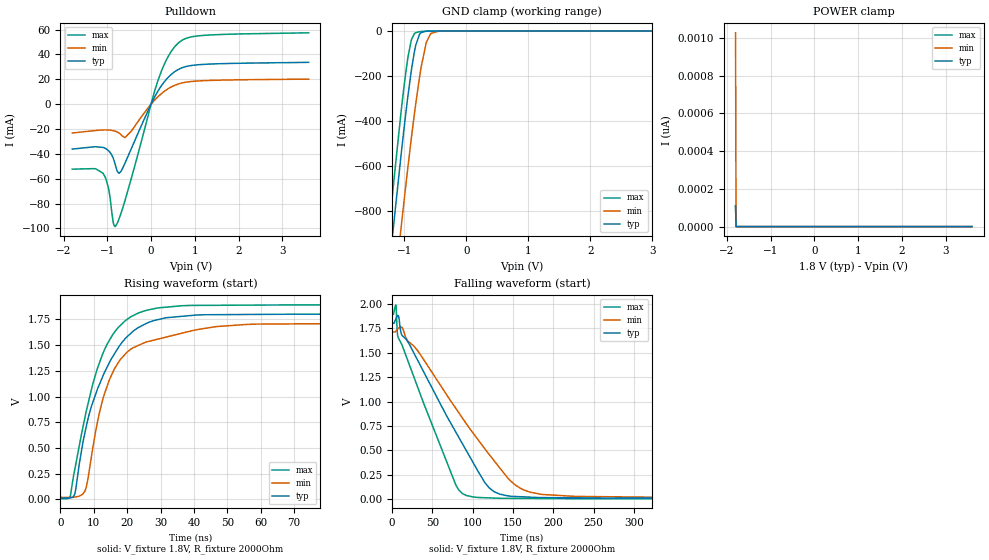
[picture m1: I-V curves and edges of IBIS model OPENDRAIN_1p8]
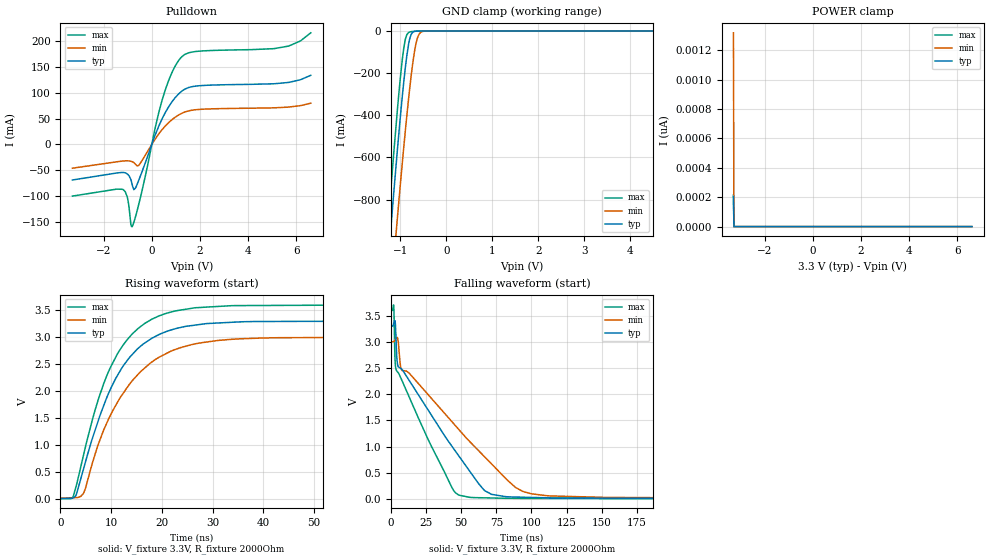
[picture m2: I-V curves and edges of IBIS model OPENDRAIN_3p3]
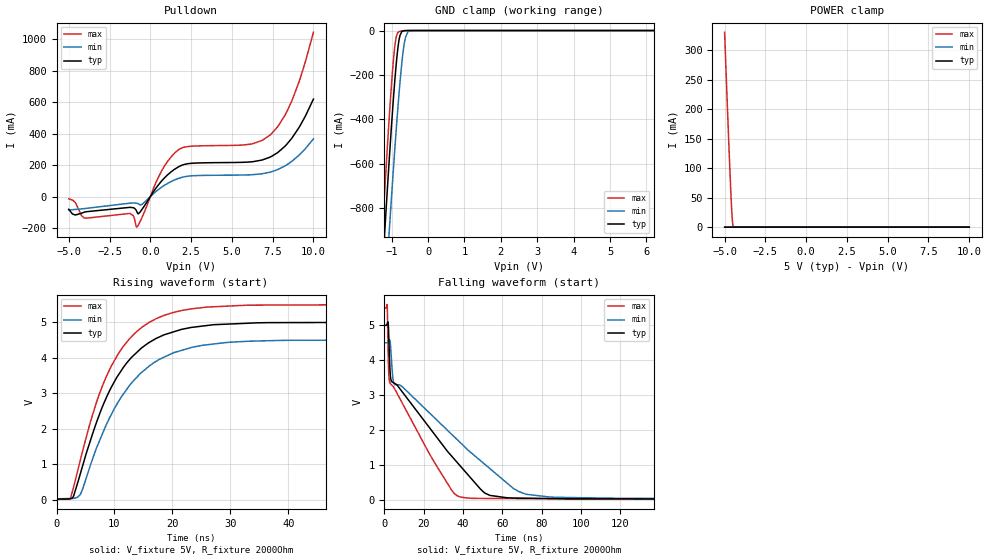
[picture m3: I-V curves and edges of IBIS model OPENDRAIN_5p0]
|Texas Instruments Incorporated
|DACx3204, Quad, 12-Bit, 10-Bit or 8-Bit, I2C Interface, Voltage/Current Output
|DACs in Tiny 3 * 3 QFN Package
[IBIS Ver]   4.1
[File name]   dac53204.ibs
[Date]   11/17/2021
[File Rev]   1.0
[Source]
| Texas Instruments Incorporated.
| Analog-eLab Design Center, HPA
| 12500 TI Blvd
| Dallas, TX -75243
[Notes]   Revision History:
| Rev 1.0: 11/17/2021
| - Initial version of the model
| - Model generated from simulations in SPECTRE
|   Model names with a trailing _1p8 contain the model for 1.8V operation.
|   Model names with a trailing _3p3 contain the model for 3.3V operation.
|   Model names with a trailing _5p0 contain the model for 5.0V operation.
| - C_comp although listed in numerical order of value are
|   obtained from varying PVT conditions. For PVT conditions for
|   each specific value refer the buffer description under
|   respective [Model]. IBIS model user is responsible for using
|   appropriate C_comp to simulate for Signal Integrity.
| - Warnings regarding combined Non-monotonicity of various models
|   have been reviewed and considered minor and can be ignored.
[Disclaimer]
| This model is designed as an aid for customers of Texas Instruments.
| TI and its licensors and suppliers make no warranties, either expressed
| or implied, with respect to this  model, including the warranties of
| merchantability or fitness for a particular purpose. The model is
| provided solely on an "as is" basis. The entire risk as to its quality
| and performance is with the customer.
| This model is subject to change without notice. Texas Instruments
| Incorporated is not responsible for updating this model.
[Copyright]
(C) Copyright 2018 Texas Instruments Incorporated.All rights reserved.
|  Component DAC53204 16-pin WQFN Package
|  Part # DAC53204
[Component]   DAC5204
[Manufacturer]  TI
[Package]   |16-pin WQFN Package
|   typ   min   max
R_pkg   0.05   0.04   0.06
L_pkg   1.0nH   0.8nH   1.2nH
C_pkg   0.2pF   0.16pF   0.24pF
[Pin]   signal_name   model_name   R_pin   L_pin   C_pin
1   FB3   NC   NA   NA   NA
2   OUT3   NC   NA   NA   NA
3   OUT2   NC   NA   NA   NA
4   FB2   NC   NA   NA   NA
5   GPIO   IO_OPENDRAIN   NA   NA   NA
6   SCL   IO_OPENDRAIN   NA   NA   NA
7   A0   IO_OPENDRAIN   NA   NA   NA
8   SDA   IO_OPENDRAIN   NA   NA   NA
9   FB1   NC   NA   NA   NA
10   OUT1   NC   NA   NA   NA
11   OUT0   NC   NA   NA   NA
12   FB0   NC   NA   NA   NA
13   CAP   NC   NA   NA   NA
14   AGND   GND   NA   NA   NA
15   VDD   POWER   NA   NA   NA
16   VREF   NC   NA   NA   NA
|   Model Selectors
[Model Selector] IO_OPENDRAIN
OPENDRAIN_1p8  1.8V   digital I/O_open_drain
OPENDRAIN_3p3  3.3V   digital I/O_open_drain
OPENDRAIN_5p0  5.0V   digital I/O_open_drain
| Models and submodels in the file (3): OPENDRAIN_1p8 (I/O_open_drain), OPENDRAIN_3p3 (I/O_open_drain), OPENDRAIN_5p0 (I/O_open_drain)
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|   OPENDRAIN_1p8 Model
[Model]   OPENDRAIN_1p8
Model_type   I/O_open_drain
Polarity   Non-Inverting
Enable   Active-Low
Vinl = 0.4
Vinh = 1.62
Vmeas = 0.9
Vref = 1.8
Cref = 2pF
Rref = 2000
|   typ   min   max
C_comp   1.258pF   1.229pF   1.287pF
[Voltage Range]   1.8   1.71   1.89
[Temperature Range]   25   125   -40
[Pullup Reference]   1.8   1.71   1.89
[Pulldown Reference]   -0   -0   0
[Power Clamp Reference]   1.8   1.71   1.89
[GND Clamp Reference]   0   0   0
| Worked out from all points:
|   slope of the pulldown table from 0 to 0.27 V, typ, clamps not added: 16.4 ohm
|   GND clamp passes 1 mA (typ) near -0.65 V on its own axis
|   falling waveform, V_fixture 1.8V, R_fixture 2000Ohm: 20-80 % time 70.5ns typ, 86.4ns min, 52.5ns max; typ from 1.8 V to 0.012 V
|   rising waveform, V_fixture 1.8V, R_fixture 2000Ohm: 20-80 % time 10.9ns typ, 9.29ns min, 9.24ns max; typ from 0.012 V to 1.8 V
[Pulldown]
|   Voltage   I(typ)   I(min)   I(max)
-1.8V     -36.15mA   -23.22mA   -52.32mA
-1.098V   -34.82mA   -20.75mA   -55.58mA
-979.2mV  -37.21mA   -20.78mA   -66.6mA
-865.8mV  -43.37mA   -21.34mA   -94.86mA
-817.2mV  -48.87mA   -21.79mA   -98.5mA
-682.2mV  -53.81mA   -24.75mA   -87.4mA
-444.6mV  -35.27mA   -21.46mA   -58.93mA
160.2mV   10.68mA    6.088mA    19.27mA
387mV     21.43mA    12.35mA    38.11mA
613.8mV   27.79mA    16.14mA    48.97mA
1.143V    31.91mA    18.82mA    55.22mA
3.6V      33.67mA    20.17mA    57.45mA
[GND Clamp]
|   Voltage   I(typ)   I(min)   I(max)
-1.8V     -2.596A    -2.851A    -2.471A
-1.433V   -1.564A    -1.858A    -1.402A
-1.201V   -928.8mA   -1.245A    -744.2mA
-1.179V   -871.1mA   -1.189A    -684.9mA
-1.055V   -548.9mA   -872.2mA   -358.3mA
-941.4mV  -281.8mA   -596mA     -112.3mA
-882mV    -162.3mA   -459.7mA   -34.2mA
-822.6mV  -68.79mA   -332mA     -7.838mA
-757.8mV  -15.19mA   -206.4mA   -2.984mA
-644.4mV  -611.1uA   -48.59mA   -607.3uA
-444.6mV  -4.804uA   -314.9uA   -3.221uA
3.6V      0A         0A         0A
[POWER Clamp]
|   Voltage   I(typ)   I(min)   I(max)
-1.8V     109.3pA    1.028nA    111pA
-1.789V   0A         0A         0A
-1.784V   0A         0A         0A
3.6V      0A         0A         0A
[Ramp]
R_load = 2000
|   typ   min   max
dV/dt_r   1.07282/1.08624e-08   1.01393/9.23116e-09   1.12988/9.2542e-09
dV/dt_f   1.07282/7.03748e-08   1.01391/8.57477e-08   1.12988/5.24625e-08
[Falling Waveform]
V_fixture = 1.8V
V_fixture_min = 1.71V
V_fixture_max = 1.89V
R_fixture = 2000Ohm
C_fixture = 0F
|   Time   V(typ)   V(min)   V(max)
0s        1.8V       1.71V      1.89V
4.646ns   1.845V     1.719V     1.988V
7.422ns   1.879V     1.748V     1.657V
12.07ns   1.68V      1.76V      1.583V
78.53ns   695.1mV    936.2mV    158mV
100.3ns   378.8mV    679.9mV    24.79mV
120.3ns   118.6mV    459.6mV    15.15mV
152.8ns   29.52mV    146.2mV    10.18mV
226.9ns   15.67mV    30.27mV    7.485mV
1.5us     11.97mV    20.15mV    6.861mV
[Rising Waveform]
V_fixture = 1.8V
V_fixture_min = 1.71V
V_fixture_max = 1.89V
R_fixture = 2000Ohm
C_fixture = 0F
|   Time   V(typ)   V(min)   V(max)
0s        11.96mV    20.12mV    6.859mV
2.913ns   14.36mV    20.15mV    27.5mV
4.236ns   47.13mV    22.99mV    281.4mV
7.365ns   652.5mV    83.69mV    800.3mV
11.76ns   1.124V     853.2mV    1.334V
15.61ns   1.385V     1.23V      1.598V
23.2ns    1.668V     1.494V     1.809V
36.28ns   1.779V     1.614V     1.882V
90.43ns   1.8V       1.71V      1.89V
1.5us     1.8V       1.71V      1.89V
|   OPENDRAIN_3p3 Model
[Model]   OPENDRAIN_3p3
Model_type   I/O_open_drain
Polarity   Non-Inverting
Enable   Active-Low
Vinl = 0.4
Vinh = 1.62
Vmeas = 1.65
Vref = 3.3
Cref = 2pF
Rref = 2000
|   typ   min   max
C_comp   1.131pF   1.106pF   1.153pF
[Voltage Range]   3.3   3   3.6
[Temperature Range]   25   125   -40
[Pullup Reference]   3.3   3   3.6
[Pulldown Reference]   0   -0   0
[Power Clamp Reference]   3.3   3   3.6
[GND Clamp Reference]   0   0   0
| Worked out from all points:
|   slope of the pulldown table from 0 to 0.495 V, typ, clamps not added: 8.87 ohm
|   GND clamp passes 1 mA (typ) near -0.66 V on its own axis
|   falling waveform, V_fixture 3.3V, R_fixture 2000Ohm: 20-80 % time 48.1ns typ, 60.7ns min, 31.5ns max; typ from 3.3 V to 0.012 V
|   rising waveform, V_fixture 3.3V, R_fixture 2000Ohm: 20-80 % time 8.9ns typ, 10.2ns min, 8.24ns max; typ from 0.012 V to 3.3 V
[Pulldown]
|   Voltage   I(typ)   I(min)   I(max)
-3.3V     -69.1mA    -46.26mA   -100.3mA
-1.191V   -54.48mA   -32.27mA   -87.74mA
-1.013V   -57.52mA   -31.89mA   -103.3mA
-874.5mV  -67.87mA   -32.75mA   -153.5mA
-815.1mV  -78.37mA   -33.62mA   -159.4mA
-745.8mV  -87.88mA   -35.39mA   -151mA
-537.9mV  -68.99mA   -40.46mA   -115.3mA
432.3mV   50.04mA    28.78mA    86.43mA
848.1mV   83.21mA    48.26mA    140.4mA
1.195V    101.2mA    59.03mA    167.3mA
5.669V    119.9mA    72.15mA    190.4mA
6.6V      133.8mA    79.76mA    216.2mA
[GND Clamp]
|   Voltage   I(typ)   I(min)   I(max)
-3.3V     -6.897A    -6.981A    -6.923A
-1.33V    -1.28A     -1.584A    -1.107A
-1.241V   -1.037A    -1.35A     -855.9mA
-1.211V   -957mA     -1.272A    -773.2mA
-1.142V   -772.7mA   -1.093A    -583.9mA
-1.063V   -568.5mA   -891.7mA   -377.7mA
-924mV    -244.9mA   -555.3mA   -84.05mA
-884.4mV  -166.7mA   -465.1mA   -36.27mA
-805.2mV  -48.92mA   -296.7mA   -5.651mA
-656.7mV  -831uA     -60.15mA   -749.1uA
-498.3mV  -21.67uA   -1.403mA   -21.19uA
6.6V      0A         0A         0A
[POWER Clamp]
|   Voltage   I(typ)   I(min)   I(max)
-3.3V     204.8pA    1.318nA    216pA
-3.28V    0A         0A         0A
-3.27V    0A         0A         0A
6.6V      0A         0A         0A
[Ramp]
R_load = 2000
|   typ   min   max
dV/dt_r   1.97274/8.89396e-09   1.78838/1.01436e-08   2.15555/8.24733e-09
dV/dt_f   1.97274/4.8229e-08   1.78837/6.07015e-08   2.15555/3.13876e-08
[Falling Waveform]
V_fixture = 3.3V
V_fixture_min = 3V
V_fixture_max = 3.6V
R_fixture = 2000Ohm
C_fixture = 0F
|   Time   V(typ)   V(min)   V(max)
0s        3.3V       3V         3.6V
1.935ns   3.349V     3.002V     3.699V
2.844ns   3.401V     3.038V     2.691V
3.754ns   2.936V     3.077V     2.462V
7.721ns   2.475V     2.456V     2.267V
43.22ns   1.014V     1.481V     227.2mV
56.02ns   532.9mV    1.098V     33.18mV
71.61ns   90.54mV    670.1mV    21.03mV
113.6ns   22.92mV    59.8mV     11.7mV
1.5us     12.11mV    19.38mV    7.413mV
[Rising Waveform]
V_fixture = 3.3V
V_fixture_min = 3V
V_fixture_max = 3.6V
R_fixture = 2000Ohm
C_fixture = 0F
|   Time   V(typ)   V(min)   V(max)
0s        12.1mV     19.37mV    7.412mV
2.481ns   22.89mV    25.66mV    40.06mV
3.1ns     77.53mV    27.23mV    241mV
4.531ns   552.1mV    105mV      808mV
6.829ns   1.276V     829.7mV    1.65V
8.915ns   1.828V     1.362V     2.234V
14.13ns   2.678V     2.19V      3.059V
21.81ns   3.135V     2.743V     3.468V
33.88ns   3.278V     2.963V     3.587V
1.5us     3.3V       3V         3.6V
|   OPENDRAIN_5p0 Model
[Model]   OPENDRAIN_5p0
Model_type   I/O_open_drain
Polarity   Non-Inverting
Enable   Active-Low
Vinl = 0.4
Vinh = 1.62
Vmeas = 2.5
Vref = 5
Cref = 2pF
Rref = 2000
|   typ   min   max
C_comp   1.041pF   1.018pF   1.056pF
[Voltage Range]   5   4.5   5.5
[Temperature Range]   25   125   -40
[Pullup Reference]   5   4.5   5.5
[Pulldown Reference]   -0   -0   0
[Power Clamp Reference]   5   4.5   5.5
[GND Clamp Reference]   0   0   0
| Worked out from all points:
|   slope of the pulldown table from 0 to 0.75 V, typ, clamps not added: 7.08 ohm
|   GND clamp passes 1 mA (typ) near -0.66 V on its own axis
|   falling waveform, V_fixture 5V, R_fixture 2000Ohm: 20-80 % time 35.2ns typ, 49ns min, 23.2ns max; typ from 5 V to 0.015 V
|   rising waveform, V_fixture 5V, R_fixture 2000Ohm: 20-80 % time 8.29ns typ, 9.08ns min, 7.85ns max; typ from 0.015 V to 5 V
[Pulldown]
|   Voltage   I(typ)   I(min)   I(max)
-5V       -80.51mA   -84.93mA   -14.22mA
-4.61V    -116.6mA   -81.76mA   -36.26mA
-4.055V   -99.11mA   -76.39mA   -136.3mA
-1.25V    -68.27mA   -41.68mA   -106.9mA
-815mV    -98.03mA   -42.8mA    -193.3mA
-545mV    -86.42mA   -51.89mA   -140.3mA
640mV     92.99mA    55.98mA    152.9mA
1.69V     186.9mA    114.2mA    294.7mA
6.115V    220.5mA    138.6mA    333.3mA
7.405V    254mA      157.2mA    397.4mA
8.68V     372mA      224.5mA    609.6mA
10V       619.9mA    367mA      1.044A
[GND Clamp]
|   Voltage   I(typ)   I(min)   I(max)
-5V       -11.57A    -11.14A    -12.21A
-1.25V    -1.062A    -1.374A    -881.6mA
-1.145V   -781.1mA   -1.101A    -592.5mA
-1.07V    -587.2mA   -910.3mA   -396.2mA
-980mV    -368.2mA   -688.1mA   -186.4mA
-920mV    -236.6mA   -546.1mA   -78.11mA
-860mV    -123.7mA   -411.3mA   -19.48mA
-785mV    -31mA      -257mA     -4.18mA
-710mV    -3.686mA   -127.3mA   -1.659mA
-650mV    -701.8uA   -53.65mA   -668.9uA
-515mV    -32.95uA   -2.223mA   -35.21uA
10V       0A         0A         0A
[POWER Clamp]
|   Voltage   I(typ)   I(min)   I(max)
-5V       960nA      3.539nA    330.6mA
-4.865V   0A         0A         231mA
-4.76V    0A         0A         155.3mA
-4.67V    0A         0A         93.19mA
-4.61V    0A         0A         54.75mA
-4.565V   0A         0A         29.41mA
-4.535V   0A         0A         15.78mA
-4.52V    0A         0A         10.49mA
-4.49V    0A         0A         3.647mA
-4.445V   0A         0A         475.5uA
10V       0A         0A         0A
[Ramp]
R_load = 2000
|   typ   min   max
dV/dt_r   2.99117/8.3009e-09   2.68662/9.05727e-09   3.29428/7.85179e-09
dV/dt_f   2.99117/3.50324e-08   2.68662/4.86741e-08   3.29428/2.31908e-08
[Falling Waveform]
V_fixture = 5V
V_fixture_min = 4.5V
V_fixture_max = 5.5V
R_fixture = 2000Ohm
C_fixture = 0F
|   Time   V(typ)   V(min)   V(max)
0s        5V         4.5V       5.5V
1.387ns   5.043V     4.501V     5.585V
2.1ns     4.854V     4.557V     3.728V
2.885ns   3.649V     4.525V     3.338V
5.106ns   3.337V     3.305V     3.189V
34.18ns   1.248V     1.874V     270.8mV
42.99ns   679.5mV    1.397V     42.9mV
68.41ns   44.68mV    230.2mV    30.29mV
87.6ns    29.31mV    66.99mV    25.05mV
1.5us     14.72mV    22.29mV    9.53mV
[Rising Waveform]
V_fixture = 5V
V_fixture_min = 4.5V
V_fixture_max = 5.5V
R_fixture = 2000Ohm
C_fixture = 0F
|   Time   V(typ)   V(min)   V(max)
0s        14.72mV    22.29mV    9.53mV
2.423ns   24.56mV    31.49mV    54.26mV
4.07ns    708.2mV    134.5mV    1.092V
5.834ns   1.659V     962.2mV    2.181V
8.301ns   2.765V     2.002V     3.356V
10.66ns   3.51V      2.757V     4.11V
13.6ns    4.111V     3.404V     4.703V
20.24ns   4.731V     4.142V     5.278V
32.93ns   4.971V     4.462V     5.481V
1.5us     5V         4.5V       5.5V
